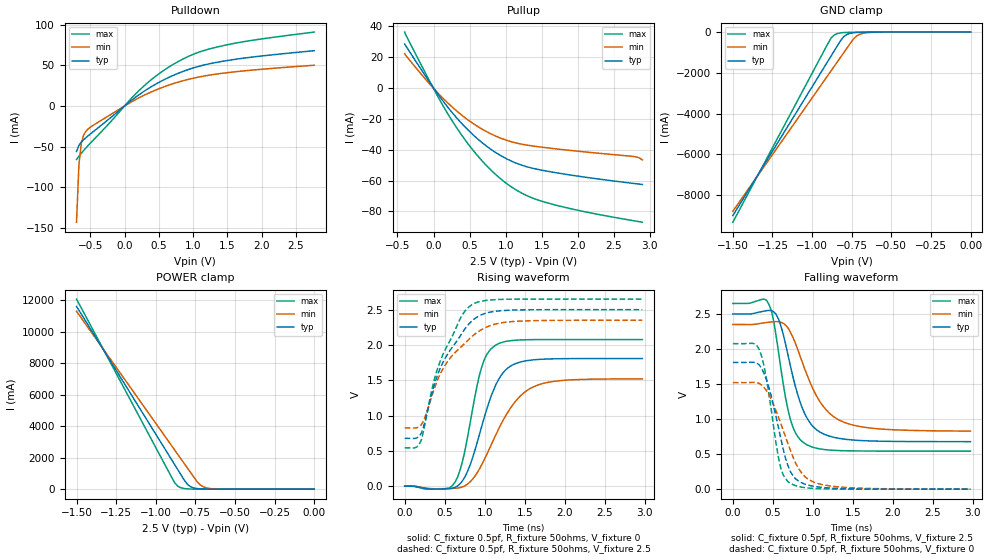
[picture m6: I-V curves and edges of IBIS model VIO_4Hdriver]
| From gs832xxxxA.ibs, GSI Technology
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|  signals   DQA1-DQA9, DQB1-DQB9, DQC1-DQC9, DQD1-DQD9
[Model]   VIO_4Hdriver
Model_type   I/O
Polarity   Non-Inverting
Vinl  =   0.75v
Vinh  =   1.75v
Vmeas =   1.25v
Cref  =   0pF
Rref  =   50
Vref  =   1.25v
|  variable   typ   min   max
C_comp   3.0pF   2.5pF   3.5pF
|  variable   typ   min   max
[Temperature Range]   50   0   100
|  variable   typ   min   max
[Voltage Range]   2.5   2.35   2.65
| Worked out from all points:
|   slope of the pulldown table from 0 to 0.375 V, typ, clamps not added: 16.4 ohm
|   slope of the pullup table from 0 to 0.375 V, typ, clamps not added: 16.9 ohm
|   GND clamp passes 1 mA (typ) near -0.58 V on its own axis
|   POWER clamp passes 1 mA (typ) near -0.61 V on its own axis
|   rising waveform, C_fixture 0.5pf, R_fixture 50ohms, V_fixture 0: 20-80 % time 307ps typ, 433ps min, 221ps max; typ from 0 V to 1.81 V
|   rising waveform, C_fixture 0.5pf, R_fixture 50ohms, V_fixture 2.5: 20-80 % time 418ps typ, 471ps min, 370ps max; typ from 0.678 V to 2.5 V
|   falling waveform, C_fixture 0.5pf, R_fixture 50ohms, V_fixture 2.5: 20-80 % time 269ps typ, 373ps min, 193ps max; typ from 2.5 V to 0.678 V
|   falling waveform, C_fixture 0.5pf, R_fixture 50ohms, V_fixture 0: 20-80 % time 230ps typ, 312ps min, 171ps max; typ from 1.81 V to 0 V
[Pulldown]
| voltage   typ   min   max
-700mV    -55.95mA   -143.1mA   -65.83mA
-665mV    -48.57mA   -71.8mA    -61.91mA
-630mV    -44.5mA    -45.69mA   -58.2mA
-595mV    -41.47mA   -35.46mA   -54.68mA
-560mV    -38.83mA   -30.72mA   -51.33mA
-490mV    -33.95mA   -25.67mA   -45.04mA
280mV     17.83mA    12.99mA    24.39mA
560mV     31.65mA    23.12mA    43.12mA
875mV     43.22mA    31.58mA    58.76mA
1.155V    50.38mA    36.79mA    68.21mA
1.54V     56.52mA    41.4mA     76.1mA
2.765V    68.04mA    50.21mA    90.98mA
[Pullup]
| voltage (VDDQ-Vout) typ   min   max
-400mV    28.37mA    22.19mA    36.15mA
25mV      -1.684mA   -1.543mA   -2.625mA
305mV     -18.57mA   -14.3mA    -24.69mA
445mV     -25.69mA   -19.59mA   -34.12mA
620mV     -33.38mA   -25.2mA    -44.44mA
795mV     -39.75mA   -29.74mA   -53.17mA
970mV     -44.85mA   -33.21mA   -60.37mA
1.25V     -50.46mA   -36.68mA   -68.78mA
1.53V     -53.53mA   -38.54mA   -73.8mA
2.055V    -57.5mA    -41.25mA   -79.77mA
2.755V    -61.75mA   -44.32mA   -85.86mA
2.895V    -62.54mA   -46.64mA   -86.96mA
[GND Clamp]
| voltage   typ   min   max
-1.5V     -9.007A    -8.796A    -9.334A
-900mV    -1.426A    -2.122A    -562.9mA
-880mV    -1.174A    -1.9A      -292.9mA
-860mV    -921.1mA   -1.678A    -142.5mA
-820mV    -416.2mA   -1.233A    -38.58mA
-800mV    -222mA     -1.011A    -23.51mA
-780mV    -116.3mA   -788.8mA   -16.2mA
-740mV    -33.04mA   -348.7mA   -9.876mA
-720mV    -18.57mA   -198.2mA   -8.142mA
-680mV    -6.87mA    -61.92mA   -5.539mA
-580mV    -1.002mA   -3.885mA   -1.438mA
0V        -366.2pA   -952.1pA   -462.1pA
[POWER Clamp]
| voltage (VDDQ-Vout) typ   min   max
-1.5V     11.62A     11.31A     12.09A
-900mV    1.877A     2.768A     763.5mA
-880mV    1.553A     2.483A     398.4mA
-860mV    1.228A     2.198A     183.4mA
-840mV    903.6mA    1.913A     83.63mA
-800mV    304.2mA    1.344A     19.44mA
-780mV    154.7mA    1.059A     10.68mA
-740mV    39.51mA    489.9mA    4.639mA
-720mV    20.32mA    274.5mA    3.532mA
-680mV    5.894mA    82.85mA    2.298mA
-580mV    568.7uA    4.201mA    684.1uA
0V        773.5pA    2.256nA    488.4pA
[Ramp]
| voltage   typ   min   max
dV/dt_r   1.53/137p   1.35/170p   1.77/112p
dV/dt_f   1.51/136p   1.31/167p   1.77/112p
R_load  =   50ohms
[Rising Waveform]
C_fixture =   0.5pf
R_fixture =   50ohms
V_fixture =   0
| Time   V(typ)   V(min)   V(max)
0s        5.712nV    13.22nV    3.887nV
510ps     -36.21mV   -33.7mV    -36.31mV
630ps     -15.86mV   -28.86mV   58.71mV
720ps     72.97mV    -10.31mV   341.5mV
780ps     196.4mV    25.53mV    661.7mV
960ps     838.4mV    298.6mV    1.678V
1.14ns    1.44V      731.7mV    2V
1.38ns    1.734V     1.196V     2.067V
1.68ns    1.796V     1.439V     2.076V
2.97ns    1.808V     1.52V      2.077V
[Rising Waveform]
C_fixture =   0.5pf
R_fixture =   50ohms
V_fixture =   2.5
V_fixture_min =   2.35
V_fixture_max =   2.65
| Time   V(typ)   V(min)   V(max)
0s        678mV      826.7mV    543.2mV
150ps     683mV      827.6mV    553.9mV
210ps     755.9mV    872.9mV    661.3mV
360ps     1.399V     1.349V     1.466V
450ps     1.687V     1.603V     1.788V
720ps     2.173V     1.99V      2.426V
840ps     2.34V      2.12V      2.57V
1.02ns    2.452V     2.252V     2.631V
1.29ns    2.491V     2.326V     2.648V
2.97ns    2.5V       2.35V      2.65V
[Falling Waveform]
C_fixture =   0.5pf
R_fixture =   50ohms
V_fixture =   2.5
V_fixture_min =   2.35
V_fixture_max =   2.65
| Time   V(typ)   V(min)   V(max)
0s        2.5V       2.35V      2.65V
450ps     2.551V     2.382V     2.639V
510ps     2.532V     2.389V     2.4V
570ps     2.429V     2.39V      1.96V
660ps     2.062V     2.34V      1.295V
720ps     1.754V     2.239V     991.9mV
900ps     1.073V     1.71V      650.8mV
1.11ns    801.9mV    1.212V     571mV
1.38ns    715.9mV    958.9mV    548.8mV
2.97ns    678.3mV    829mV      543.3mV
[Falling Waveform]
C_fixture =   0.5pf
R_fixture =   50ohms
V_fixture =   0
| Time   V(typ)   V(min)   V(max)
0s        1.808V     1.52V      2.077V
330ps     1.772V     1.509V     1.993V
390ps     1.649V     1.451V     1.755V
450ps     1.45V      1.346V     1.361V
540ps     1.033V     1.117V     648.4mV
600ps     718.7mV    932.9mV    293.8mV
720ps     248.5mV    551mV      82mV
870ps     85.15mV    216mV      27.3mV
1.11ns    26.13mV    66.95mV    5.338mV
2.97ns    10.37uV    274.4uV    233.3nV
